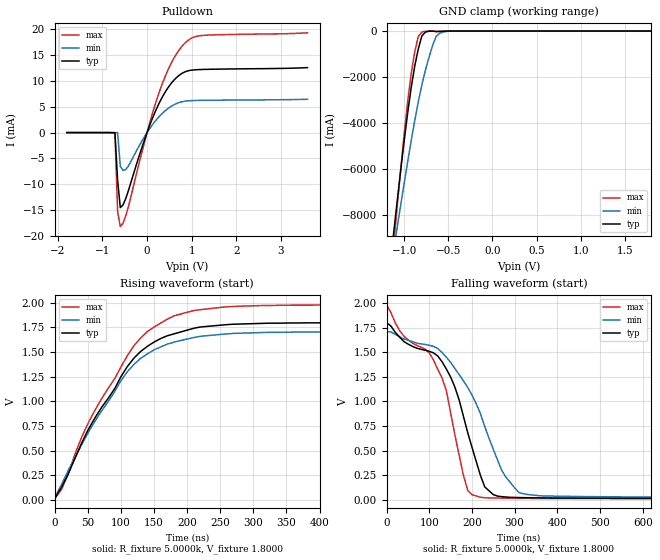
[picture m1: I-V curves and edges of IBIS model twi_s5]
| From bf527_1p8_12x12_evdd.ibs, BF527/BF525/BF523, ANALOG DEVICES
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|   Model ptwi400kv123
[Model]   twi_s5
Model_type I/O_open_drain
Polarity   Non-Inverting
Enable   Active-Low
Vinl =   0.5400V
Vinh =   1.2600V
Vmeas =  0.9000V
Cref =   50.0000pF
Rref =   5.0000k
Vref =   1.8000V
C_comp   7.1300pF   6.4200pF   7.8500pF
[Temperature Range]   25.0000   0.1250k   0.0
[Voltage Range]   1.8000V   1.7100V   1.9800V
[Pullup Reference]   1.8000V   1.7100V   1.9800V
[Pulldown Reference]   0.0V   0.0V   0.0V
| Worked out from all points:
|   slope of the pulldown table from 0 to 0.27 V, typ, clamps not added: 47.9 ohm
|   GND clamp passes 1 mA (typ) near -0.44 V on its own axis
|   rising waveform, R_fixture 5.0000k, V_fixture 1.8000: 20-80 % time 92.7ns typ, 94ns min, 94.7ns max; typ from 0.015 V to 1.8 V
|   falling waveform, R_fixture 5.0000k, V_fixture 1.8000: 20-80 % time 88.2ns typ, 110ns min, 109ns max; typ from 1.8 V to 0.015 V
[Pulldown]
|Voltage   I(typ)   I(min)   I(max)
-1.8V     0A         0A         0A
-720mV    -20uA      0A         -63uA
-660mV    -9.21mA    0A         -15.24mA
-600mV    -14.49mA   -6.5mA     -18.15mA
-480mV    -12.81mA   -7.167mA   -16.15mA
0V        0A         0A         0A
300mV     6.168mA    3.352mA    8.441mA
600mV     10.1mA     5.361mA    14.33mA
840mV     11.69mA    6.059mA    17.21mA
1.02V     12.08mA    6.188mA    18.34mA
1.26V     12.2mA     6.231mA    18.77mA
3.6V      12.55mA    6.443mA    19.27mA
[GND_clamp]
|Voltage   I(typ)   I(min)   I(max)
-1.8V     -33.68A    -27.13A    -39.84A
-1.12V    -8.799A    -9.55A     -9.344A
-1.08V    -7.418A    -8.558A    -7.664A
-1V       -4.765A    -6.614A    -4.473A
-920mV    -2.435A    -4.756A    -1.824A
-880mV    -1.51A     -3.883A    -890.2mA
-840mV    -771.5mA   -3.07A     -231.1mA
-800mV    -213.7mA   -2.34A     -43.87mA
-720mV    -10.17mA   -1.149A    -2.199mA
-640mV    -19.29mA   -242.9mA   -27.34mA
-560mV    -8.563mA   -41mA      -13.65mA
1.8V      437.9pA    17.59nA    412.5pA
[Ramp]
| variable   typ   min   max
dV/dt_r  1.0705/92.9931n   1.0102/94.2758n   1.1801/94.9346n
dV/dt_f  1.0710/88.1758n   1.0096/0.1100u   1.1806/0.1096u
R_load = 5.0000k
[Rising Waveform]
R_fixture= 5.0000k
V_fixture= 1.8000
V_fixture_min= 1.7100
V_fixture_max= 1.9800
L_fixture= 0.0H
C_fixture= 0.0F
|time   V(typ)   V(min)   V(max)
0s        14.79mV    25.39mV    12.21mV
10.1ns    127.4mV    154.4mV    104.9mV
40.4ns    573.7mV    557.5mV    633.4mV
50.51ns   712.7mV    683.1mV    780.3mV
110ns     1.357V     1.304V     1.468V
140ns     1.559V     1.483V     1.709V
180ns     1.685V     1.601V     1.868V
220ns     1.755V     1.661V     1.931V
320ns     1.793V     1.7V       1.973V
1us       1.799V     1.709V     1.979V
[Falling Waveform]
R_fixture= 5.0000k
V_fixture= 1.8000
V_fixture_min= 1.7100
V_fixture_max= 1.9800
L_fixture= 0.0H
C_fixture= 0.0F
|time   V(typ)   V(min)   V(max)
0s        1.8V       1.709V     1.98V
30.3ns    1.655V     1.656V     1.721V
100ns     1.509V     1.57V      1.494V
130ns     1.402V     1.496V     1.237V
180ns     849mV      1.209V     248.6mV
200ns     535.2mV    1.065V     52.82mV
230ns     131.5mV    744.2mV    21.78mV
270ns     32.91mV    297.6mV    18.02mV
310ns     23.87mV    74.7mV     15.87mV
1us       15.03mV    26.25mV    12.27mV
